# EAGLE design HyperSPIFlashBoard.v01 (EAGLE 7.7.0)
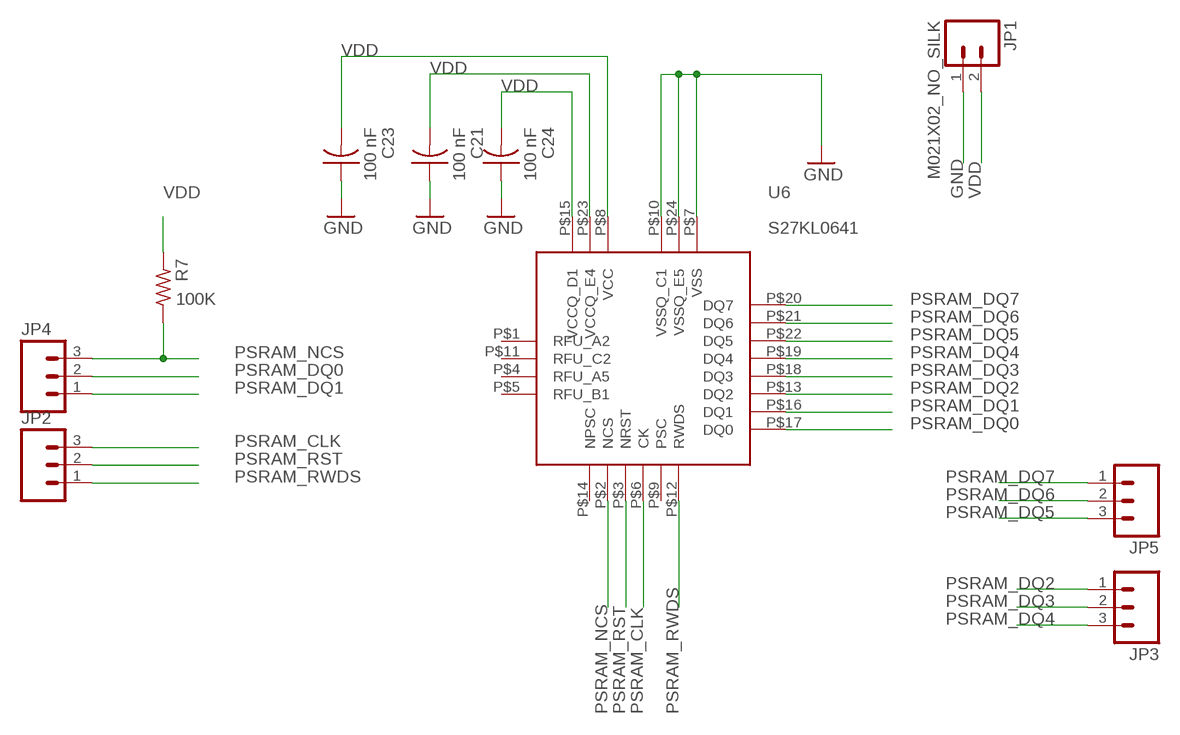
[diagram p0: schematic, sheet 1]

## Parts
C21  100 nF  C-US  [C0402_B]
C23  100 nF  C-US  [C0402_B]
C24  100 nF  C-US  [C0402_B]
JP1  M021X02_NO_SILK  [1X02_NO_SILK]
JP2  M031X03_NO_SILK  [1X03_NO_SILK]
JP3  M031X03_NO_SILK  [1X03_NO_SILK]
JP4  M031X03_NO_SILK  [1X03_NO_SILK]
JP5  M031X03_NO_SILK  [1X03_NO_SILK]
R7  100K  R-US_  [R0402_B]
U6  S27KL0641  [S27KL0641]

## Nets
GND: C21.1 C23.1 C24.1 JP1.1 U6.P$7(VSS) U6.P$10(VSSQ_C1) U6.P$24(VSSQ_E5)
PSRAM_CLK: JP2.3 U6.P$6(CK)
PSRAM_DQ0: JP4.2 U6.P$17(DQ0)
PSRAM_DQ1: JP4.1 U6.P$16(DQ1)
PSRAM_DQ2: JP3.1 U6.P$13(DQ2)
PSRAM_DQ3: JP3.2 U6.P$18(DQ3)
PSRAM_DQ4: JP3.3 U6.P$19(DQ4)
PSRAM_DQ5: JP5.3 U6.P$22(DQ5)
PSRAM_DQ6: JP5.2 U6.P$21(DQ6)
PSRAM_DQ7: JP5.1 U6.P$20(DQ7)
PSRAM_NCS: JP4.3 R7.1 U6.P$2(NCS)
PSRAM_RST: JP2.2 U6.P$3(NRST)
PSRAM_RWDS: JP2.1 U6.P$12(RWDS)
VDD: C21.2 C23.2 C24.2 JP1.2 R7.2 U6.P$8(VCC) U6.P$15(VCCQ_D1) U6.P$23(VCCQ_E4)
Unconnected: U6.P$1(RFU_A2) U6.P$4(RFU_A5) U6.P$5(RFU_B1) U6.P$9(PSC) U6.P$11(RFU_C2) U6.P$14(NPSC)

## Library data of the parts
C21 C23 C24 = Spark:C-US: Capacitor
JP1 = SparkFun-Connectors:M02: Standard 2-pin 0.1" header. Use with
JP2-JP5 = SparkFun-Connectors:M03: Header 3 Standard 3-pin 0.1" header. Use with straight break away headers (SKU : PRT-00116), right angle break away headers (PRT-00553), swiss pins (PRT-00743), machine pins (PRT-00117), and female headers (PRT-00115). Molex polarized connector foot print use with SKU : PRT-08232 with associated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
R7 = Spark:R-US_: 0402 Resistor
U6 = Kris:S27KL0641: S27KL0641 hyperRam PSRAM 64 Mbit https://www.cypress.com/file/183506/download

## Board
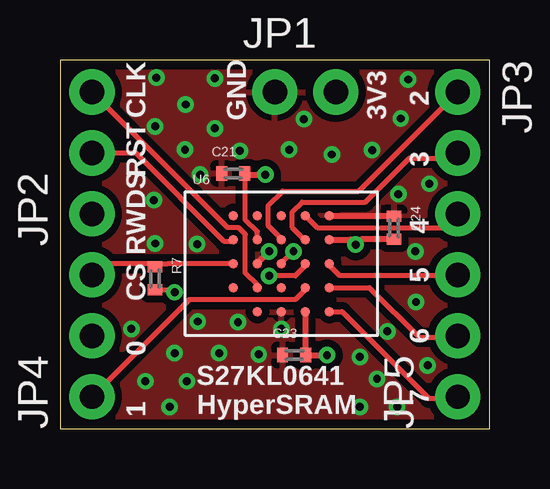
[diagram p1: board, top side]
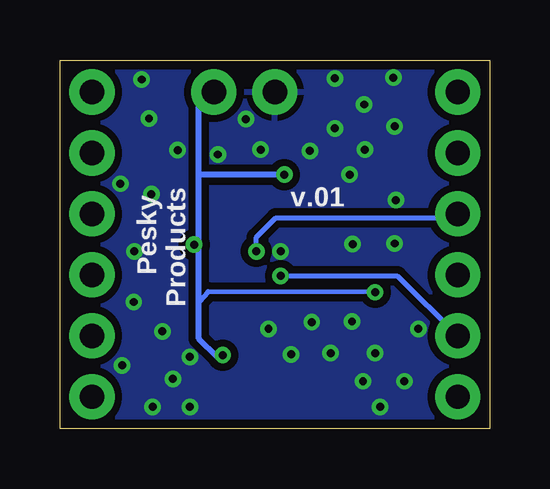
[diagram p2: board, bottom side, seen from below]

Size 17.91 x 15.37 mm. Coordinates in mm from the lower left corner, seen from the top.
Outline: 17.91,0 17.91,15.37 0,15.37 0,0 17.91,0
Copper layers (1*16): Top 0.0356mm / dielectric 1.5011mm / Bottom 0.0356mm
Design rules "oshpark-2layer *": minimum track width 6mil, minimum drill 13mil, track to track 6mil, track to pad 6mil, pad to pad 6mil, via to via 6mil, smd to smd 6mil, copper to edge 15mil, drill to drill 6mil, minimum pad ring 7mil, minimum via ring 7mil, stop-mask expansion 4mil, vias tented up to drill 20mil, thermal gap 10mil

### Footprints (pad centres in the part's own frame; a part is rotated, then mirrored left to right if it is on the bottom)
C0402_B = smd 0.457 x 0.61: 1 -0.483,0; 2 0.483,0
1X02_NO_SILK = drill 1.016 pad 1.88: 1 0,0; 2 2.54,0
1X03_NO_SILK = drill 1.016 pad 1.88: 1 0,0; 2 2.54,0; 3 5.08,0
R0402_B = smd 0.457 x 0.61: 1 -0.483,0; 2 0.483,0
S27KL0641 = smd 0.4 x 0.4: P$1 -2,-1; P$2 -2,0; P$3 -2,1; P$4 -2,2; P$5 -1,-2; P$6 -1,-1; P$7 -1,0; P$8 -1,1; P$9 -1,2; P$10 0,-2; P$11 0,-1; P$12 0,0; P$13 0,1; P$14 0,2; P$15 1,-2; P$16 1,-1; P$17 1,0; P$18 1,1; P$19 1,2; P$20 2,-2; P$21 2,-1; P$22 2,0; P$23 2,1; P$24 2,2

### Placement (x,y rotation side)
C21  7.21,10.64 0 top
C23  9.75,3.07 0 top
C24  13.92,8.38 270 top
JP1  8.95,14.03 0 top
JP2  1.33,8.95 90 top
JP3  16.57,14.03 270 top
JP4  1.33,1.33 90 top
JP5  16.57,1.33 90 top
R7  3.96,6.27 270 top
U6  9.22,6.88 0 top

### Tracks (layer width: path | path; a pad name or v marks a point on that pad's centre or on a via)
GND  (via drill 0.33)
  Top 0.254: U6.P$24 13.9,8.88 C24.1 | U6.P$7 8.22,6.9 v8.71,7.39
  other vias: 15.39,10.21 9.22,4.17 3.96,7.72 13.64,4.06 14.83,5.28 14.81,7.39 3.91,9.53 5.84,10.59 11.33,11.43 14.5,14.55 13,11.61 10.16,12.9 6.45,14.61 4.01,14.63 5.23,13.51 3.96,12.6 6.45,12.52 5.21,11.63 7.49,11.58 9.55,11.63 2.97,4.17 5.71,7.7 5.74,4.47 7.42,4.45 8.28,3.1 6.63,3.15 4.78,3.15 3.56,1.98 5.28,1.98 4.57,0.91 12.5,3 12.5,0.91 13.21,2.08 14.05,0.91 15.32,2.64 14.2,12.93 14.1,9.78
  pour Bottom (isolate 0.305): 0,15.37 0,0 17.93,0 17.93,15.37
  pour Top (isolate 0.305): 0,15.37 0,0 17.83,0 17.83,15.37
PSRAM_CLK
  Top 0.203: U6.P$6 8.22,6 7.72,6.48 7.72,8.1 7.44,8.38 6.99,8.38 JP2.3
PSRAM_DQ0  (via drill 0.33)
  Top 0.203: U6.P$17 10.22,6.79 9.8,6.38 v8.71,6.38
  Bottom 0.203: v8.71,6.38 3.86,6.38 JP4.2
PSRAM_DQ1
  Top 0.203: U6.P$16 10.22,5.8 9.8,5.38 5.38,5.38 JP4.1
PSRAM_DQ2
  Top 0.203: U6.P$13 9.22,7.92 8.69,8.46 8.69,9.32 9.27,9.91 12.45,9.91 JP3.1
PSRAM_DQ3
  Top 0.203: U6.P$18 10.18,7.88 9.68,8.38 9.68,9.04 10.08,9.45 12.72,9.45 14.55,11.28 16.36,11.28 JP3.2
PSRAM_DQ4
  Top 0.203: U6.P$19 10.72,8.38 16,8.38 JP3.3
PSRAM_DQ5
  Top 0.203: U6.P$22 11.22,6.81 11.63,6.4 JP5.3
PSRAM_DQ6
  Top 0.203: U6.P$21 12.89,5.88 14.96,3.81 16.51,3.81 JP5.2
PSRAM_DQ7
  Top 0.203: U6.P$20 11.75,4.88 15.37,1.27 16.51,1.27 JP5.1
PSRAM_NCS
  Top 0.203: U6.P$2 4.5,6.88 4.14,6.88 | 4.14,6.88 1.8,6.88 JP4.3 | R7.1 4.14,6.88
PSRAM_RST
  Top 0.203: JP2.2 3.16,11.49 6.83,7.82 7.16,7.82 U6.P$3
PSRAM_RWDS  (via drill 0.33)
  Top 0.203: U6.P$12 9.22,6.91 v9.73,7.39
  Bottom 0.203: v9.73,7.39 9.73,7.98 8.91,8.79 1.5,8.79 JP2.1
VDD  (via drill 0.33)
  Top 0.203: U6.P$8 8.22,8.21 7.72,8.69 7.72,10.52 C21.2 | R7.2 4.6,5.79 v4.78,5.69
  Top 0.254: 13.9,7.88 C24.2 12.57,7.9 v12.32,7.67 12.11,7.88 U6.P$23 | v11.12,3.07 C23.2 10.22,3.06 U6.P$15 | C21.2 7.82,10.59 v8.56,10.59
  Bottom 0.203: v4.78,5.69 11.73,5.71 12.12,5.28
  Bottom 0.254: v11.12,3.07 11.35,3 12.12,3.76 12.12,5.28 12.12,7.8 | 12.12,7.8 12.12,10.57 | 12.12,10.57 12.12,13.41 JP1.2 | v12.32,7.67 12.12,7.8 | v8.56,10.59 12.09,10.59 12.12,10.57

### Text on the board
tPlace: CLK | GND | 3V3 | 2 | 3 | RST | 4 | RWDS | 5 | CS | 6 | 0 | 1 | S27KL0641 / HyperSRAM | 7
bPlace: Pesky / Products | v.01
